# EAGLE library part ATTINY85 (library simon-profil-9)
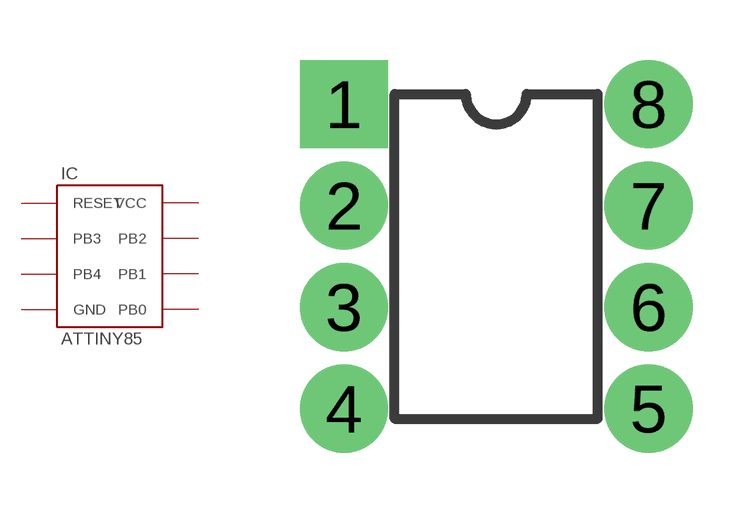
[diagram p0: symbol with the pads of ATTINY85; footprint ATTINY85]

Designator prefix IC

## ATTINY85  [ATTINY85]
1  RESET
2  PB3
3  PB4
4  GND
5  PB0
6  PB1
7  PB2
8  VCC

## Footprint ATTINY85 (pad centres in mm)
Original name ATTINY85
drill 0.914 pad 2.21 square: 1 -3.81,3.81
drill 0.914 pad 2.21: 2 -3.81,1.27; 3 -3.81,-1.27; 4 -3.81,-3.81; 5 3.81,-3.81; 6 3.81,-1.27; 7 3.81,1.27; 8 3.81,3.81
